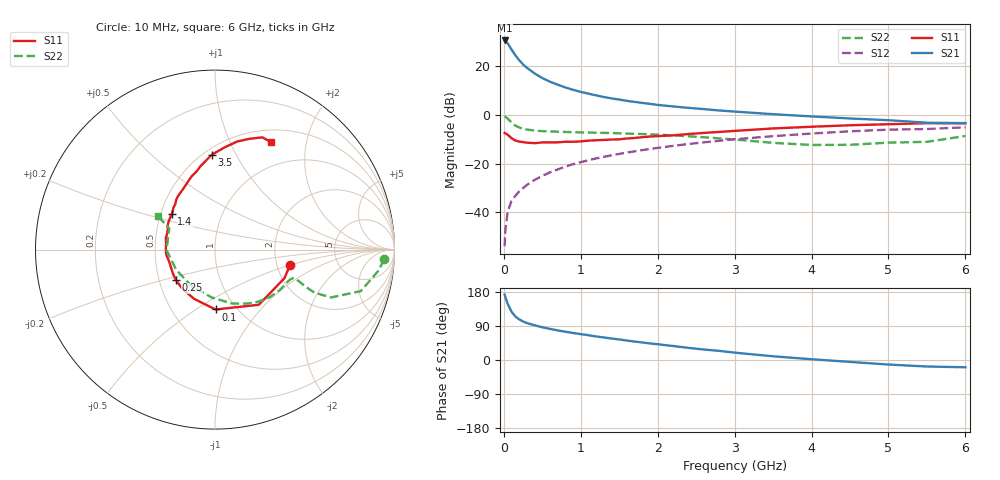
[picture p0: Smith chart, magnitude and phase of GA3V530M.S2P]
! Infineon Technologies  Discrete & RF Semiconductors
! BF775
! Si NPN RF Bipolar Junction Transistor in SOT23
! VCE = 3.5 V  IC = 30 mA
! Common Emitter S-Parameters:  May  1996
# GHz  S  MA  R  50
!  f  S11  S21  S12  S22
! GHz  MAG  ANG  MAG  ANG  MAG  ANG  MAG  ANG
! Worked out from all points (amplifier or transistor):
!   36 points, 10 MHz to 6 GHz, reference 50 ohm
!   highest |S21| = 30.7 dB at 10 MHz (marker M1)
!   |S21| within 3 dB of that: start of sweep to 85.63 MHz
!   unconditionally stable (mu >= 1): 237.6 MHz to 3.233 GHz; 5.47 GHz to 5.577 GHz
!   at 250 MHz: K = 1.02, MAG = 24.6 dB, |S12| = -30.1 dB
!   at 1.4 GHz: K = 1.17, MAG = 9.2 dB, |S12| = -16.6 dB
!   at 6 GHz: K = 0.99, MSG = 0.9 dB, |S12| = -5.1 dB
!   S11 on the Smith chart (normalised r, x): 10 MHz: 2.37, -0.48; 100 MHz: 0.80, -0.60; 250 MHz: 0.61, -0.23; 1.4 GHz: 0.57, +0.25; 3.5 GHz: 0.55, +0.80; 6 GHz: 0.66, +1.44
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0.01  0.4265 -11.3  34.23 172.8  0.002 82.2  0.9422 -3.3
0.02  0.4189 -22.2  33.62 165.8  0.0043 81.2  0.9211 -7.1
0.05  0.3926 -51.5  29.88 147.9  0.0103 75.2  0.8443 -15.9
0.1  0.3337 -89.5  22.27 127.4  0.0171 68.4  0.6996 -22.4
0.15  0.2981 -113.0  16.91 114.9  0.0218 66.6  0.6044 -23.4
0.2  0.2844 -129.3  13.42 107.2  0.0268 67.5  0.5539 -22.5
0.25  0.2766 -142.0  10.99 101.7  0.0312 69.1  0.5216 -21.5
0.3  0.2696 -150.9  9.356 97.5  0.0365 70.7  0.5028 -20.8
0.4  0.2635 -164.3  7.18 91.7  0.0462 72.2  0.4799 -20.0
0.5  0.2728 -173.7  5.76 86.3  0.0559 72.9  0.4654 -20.0
0.6  0.2742 179.3  4.848 82.1  0.0662 72.8  0.4599 -20.4
0.8  0.2814 167.0  3.692 74.7  0.0867 72.1  0.4479 -22.4
0.9  0.2813 161.4  3.302 71.3  0.0974 71.7  0.4432 -23.7
1.1  0.297 152.5  2.751 65.4  0.1175 70.5  0.4358 -26.9
1.4  0.3127 140.5  2.201 56.7  0.1482 68.0  0.4257 -31.9
1.7  0.3364 131.0  1.861 48.6  0.1788 64.9  0.4099 -37.7
2.2  0.3818 117.7  1.503 36.9  0.2318 59.4  0.3805 -49.0
3  0.4716 99.9  1.177 19.4  0.3168 49.4  0.314 -72.7
3.5  0.5291 91.9  1.04 9.8  0.3668 42.6  0.2675 -93.8
4.5  0.6154 78.3  0.849 -5.0  0.4624 28.1  0.2438 -152.5
5.5  0.6789 67.1  0.694 -17.2  0.5152 12.1  0.2806 155.2
6  0.6753 62.3  0.681 -19.2  0.5587 7.6  0.3704 149.5
